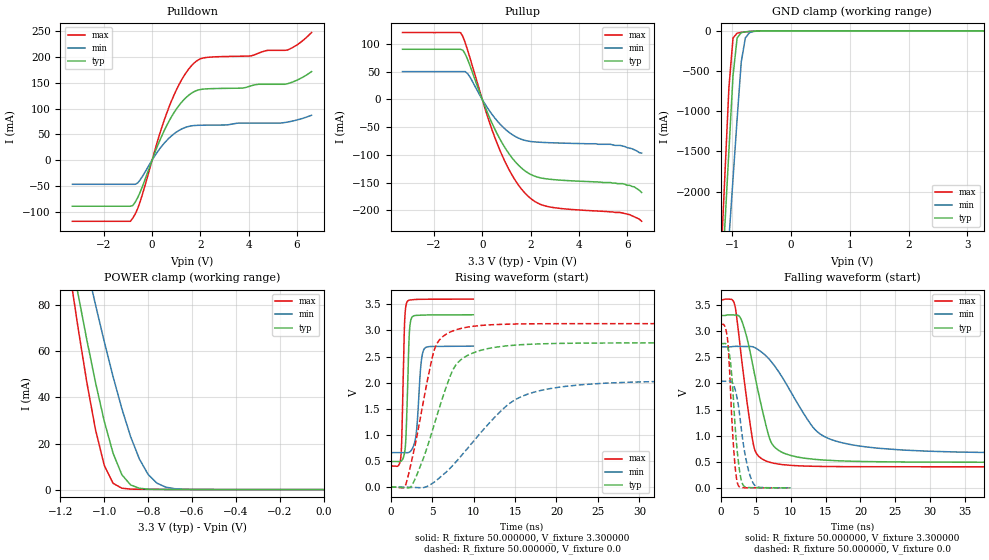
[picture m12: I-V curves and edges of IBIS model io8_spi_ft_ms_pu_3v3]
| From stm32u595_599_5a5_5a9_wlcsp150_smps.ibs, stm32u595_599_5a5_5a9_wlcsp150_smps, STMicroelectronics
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|   Model io8_spi_ft_ms_pu_3v3
[Model]  io8_spi_ft_ms_pu_3v3
Model_type I/O
Polarity   Non-Inverting
Enable   Active-Low
Vinl =   0.990000V
Vinh =   2.310000V
Vmeas =  1.650000V
Cref =   50.000000pF
Rref =   100.000000M
Vref =   0.0V
C_comp   3.495300pF   3.468500pF   3.534700pF
[Temperature Range]   25.000000   0.140000k   -40.000000
[Pullup Reference]   3.300000V   2.700000V   3.600000V
[Pulldown Reference]   0.0V   0.0V   0.0V
[POWER Clamp Reference]   3.300000V   2.700000V   3.600000V
[GND Clamp Reference]   0.0V   0.0V   0.0V
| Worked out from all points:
|   slope of the pulldown table from 0 to 0.495 V, typ, clamps not added: 8.73 ohm
|   slope of the pullup table from 0 to 0.495 V, typ, clamps not added: 9.64 ohm
|   GND clamp passes 1 mA (typ) near -0.50 V on its own axis
|   POWER clamp passes 1 mA (typ) near -0.85 V on its own axis
|   rising waveform, R_fixture 50.000000, V_fixture 3.300000: 20-80 % time 327ps typ, 511ps min, 283ps max; typ from 0.491 V to 3.3 V
|   rising waveform, R_fixture 50.000000, V_fixture 0.0: 20-80 % time 3.46ns typ, 7.17ns min, 2.35ns max; typ from 0.001 V to 2.76 V
|   falling waveform, R_fixture 50.000000, V_fixture 3.300000: 20-80 % time 2.77ns typ, 5.94ns min, 1.85ns max; typ from 3.3 V to 0.491 V
|   falling waveform, R_fixture 50.000000, V_fixture 0.0: 20-80 % time 944ps typ, 1.38ns min, 767ps max; typ from 2.76 V to 0.001 V
[Pulldown]
|Voltage   I(typ)   I(min)   I(max)
-3.3V     -89.71mA   -47.06mA   -119mA
-900mV    -89.71mA   -47.06mA   -119mA
-700mV    -81.75mA   -47.06mA   -104.8mA
-500mV    -62.92mA   -38.71mA   -81.44mA
300mV     36.2mA     21.01mA    48.7mA
800mV     84.06mA    46.96mA    114.8mA
1.3V      116.7mA    62.08mA    162.4mA
1.8V      134.4mA    67.38mA    191.2mA
2.2V      138.3mA    67.91mA    199.2mA
4.1V      144.4mA    71.94mA    202.7mA
5.6V      148.4mA    73.89mA    213.9mA
6.6V      172mA      87.1mA     247.9mA
[Pullup]
|Voltage   I(typ)   I(min)   I(max)
-3.3V     90.49mA    50.18mA    120.6mA
-900mV    90.49mA    50.18mA    120.6mA
-800mV    88.72mA    50.18mA    113.4mA
-600mV    71.49mA    46.18mA    88.08mA
200mV     -22.26mA   -14.13mA   -28.38mA
700mV     -69mA      -42.82mA   -88.5mA
1.3V      -109.1mA   -65.19mA   -141.4mA
2V        -135.3mA   -75.91mA   -178.7mA
2.9V      -144.6mA   -78.33mA   -194.9mA
5.8V      -152mA     -84mA      -205mA
6.3V      -158mA     -91mA      -212mA
6.6V      -168mA     -97mA      -220mA
[GND_clamp]
|Voltage   I(typ)   I(min)   I(max)
-3.3V     -9.098A    -9.372A    -9.671A
-1.2V     -3.386A    -4.091A    -2.933A
-1.13V    -2.437A    -3.34A     -1.815A
-1.06V    -1.49A     -2.588A    -705.6mA
-990mV    -555.7mA   -1.839A    -89.03mA
-920mV    -88.12mA   -1.093A    -28.78mA
-850mV    -22.35mA   -387.4mA   -19.84mA
-780mV    -12.12mA   -88mA      -13.87mA
-710mV    -7.709mA   -22.52mA   -8.846mA
-640mV    -4.545mA   -7.864mA   -4.87mA
-360mV    -31.12uA   -173.5uA   -8.496uA
3.28V     0A         14.15nA    -7.901nA
[POWER_clamp]
|Voltage   I(typ)   I(min)   I(max)
-3.28V    1.355A     1.167A     1.665A
-1.16V    105.8mA    131.6mA    95.87mA
-1.12V    85.08mA    114mA      70.45mA
-1.08V    65.17mA    96.88mA    46.73mA
-1.04V    46.48mA    80.2mA     25.96mA
-1V       29.63mA    64.18mA    10.49mA
-960mV    15.81mA    49.06mA    2.743mA
-920mV    6.481mA    35.16mA    612.1uA
-840mV    577.5uA    13.29mA    137.7uA
-760mV    93.74uA    2.807mA    97.79uA
-640mV    40.06uA    158.9uA    59.34uA
0V        0A         19.33nA    0A
[Ramp]
| variable   typ   min   max
dV/dt_r  1.65687/3.45088n   1.22430/7.15777n   1.87825/2.34527n
dV/dt_f  1.68568/2.76451n   1.22240/5.92981n   1.91752/1.84431n
R_load = 50.000000
[Rising Waveform]
R_fixture= 50.000000
V_fixture= 3.300000
V_fixture_min= 2.700000
V_fixture_max= 3.600000
|time   V(typ)   V(min)   V(max)
0s        490.5mV    660.4mV    404.1mV
1.241ns   494.5mV    660.4mV    584mV
1.682ns   655.8mV    660mV      3.114V
1.982ns   1.54V      659mV      3.545V
2.262ns   2.944V     669.9mV    3.581V
2.563ns   3.249V     719.8mV    3.587V
3.083ns   3.288V     1.012V     3.594V
3.644ns   3.292V     2.315V     3.597V
4.024ns   3.295V     2.639V     3.597V
9.97ns    3.3V       2.7V       3.6V
[Rising Waveform]
R_fixture= 50.000000
V_fixture= 0.0
V_fixture_min= 0.0
V_fixture_max= 0.0
|time   V(typ)   V(min)   V(max)
0s        563uV      600.6uV    581.8uV
1.682ns   -10.29mV   756.6uV    -814.3uV
2.643ns   55.43mV    -6.922mV   577.2mV
5.285ns   1.209V     99.11mV    2.638V
6.246ns   1.7V       225.9mV    2.875V
7.928ns   2.35V      491.8mV    3.015V
10.21ns   2.586V     919.5mV    3.085V
14.05ns   2.707V     1.566V     3.119V
19.1ns    2.748V     1.883V     3.129V
59.82ns   2.762V     2.041V     3.131V
[Falling Waveform]
R_fixture= 50.000000
V_fixture= 3.300000
V_fixture_min= 2.700000
V_fixture_max= 3.600000
|time   V(typ)   V(min)   V(max)
0s        3.3V       2.7V       3.6V
1.922ns   3.31V      2.709V     3.544V
3.003ns   3.203V     2.708V     2.449V
4.805ns   2.203V     2.691V     757.9mV
6.486ns   1.192V     2.527V     515.2mV
7.327ns   847mV      2.401V     480.1mV
8.889ns   674.3mV    2.1V       444.7mV
13.45ns   546.4mV    1.123V     413.2mV
17.18ns   517mV      870.2mV    407.5mV
59.82ns   490.5mV    660.4mV    404.1mV
[Falling Waveform]
R_fixture= 50.000000
V_fixture= 0.0
V_fixture_min= 0.0
V_fixture_max= 0.0
|time   V(typ)   V(min)   V(max)
0s        2.762V     2.041V     3.131V
560.6ps   2.765V     2.041V     3.101V
981ps     2.697V     2.041V     2.842V
1.421ns   2.389V     2.044V     1.801V
1.862ns   1.602V     1.964V     741.8mV
2.482ns   558.2mV    1.618V     57.54mV
3.163ns   64.12mV    912.7mV    4.824mV
3.864ns   8.187mV    397.5mV    2.437mV
4.705ns   3.368mV    78.59mV    1.592mV
9.97ns    563uV      600.6uV    581.8uV
